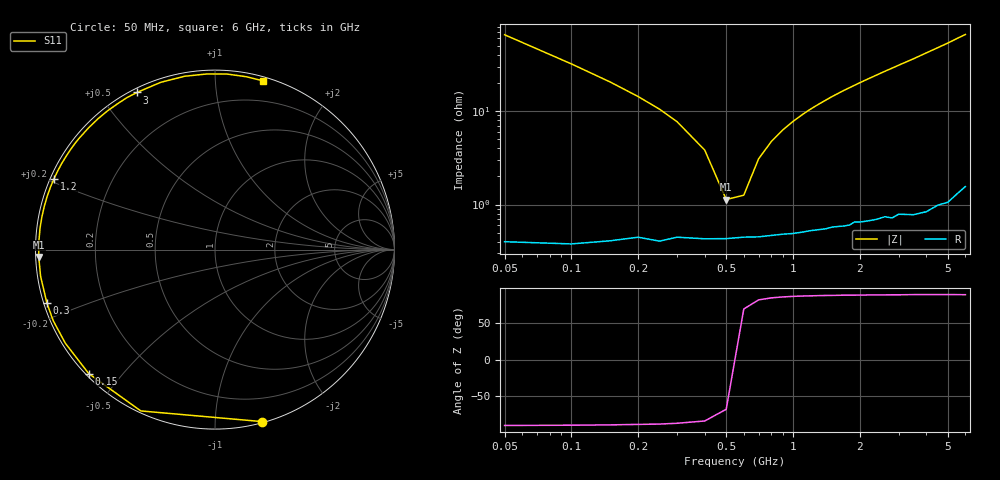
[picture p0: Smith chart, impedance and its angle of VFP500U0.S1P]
! Infineon Technologies  Discrete & RF Semiconductors
! BBY 58-03
! Si Tuning Diode in SOD323
! VR = 0.5 V
! S-Parameters:  June  1999
# GHz  S  MA  R  50
!  f  S11
! GHz  MAG  ANG
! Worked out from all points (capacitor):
!   34 points, 50 MHz to 6 GHz, reference 50 ohm
!   read as one part to ground: C = 48 pF near 50 MHz
!   lowest |Z| = 1.13 ohm at 500 MHz (marker M1)
!   series resonance near 547.1 MHz, so ESL is about 1.8 nH
!   S11 on the Smith chart (normalised r, x): 50 MHz: 0.01, -1.31; 150 MHz: 0.01, -0.41; 300 MHz: 0.01, -0.15; 1.2 GHz: 0.01, +0.21; 3 GHz: 0.02, +0.62; 6 GHz: 0.03, +1.32
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0.05  0.9941 -74.6
0.1  0.9893 -114.7
0.15  0.986 -135.5
0.2  0.9836 -148.0
0.25  0.9845 -156.3
0.3  0.9827 -162.5
0.4  0.983 -171.3
0.5  0.9829 -177.6
0.6  0.9822 177.3
0.7  0.9822 173.0
0.8  0.9816 169.2
1  0.981 162.4
1.2  0.98 156.3
1.4  0.9796 150.8
1.6  0.9789 145.6
1.7  0.979 143.1
2  0.9779 136.2
2.2  0.9778 131.9
2.4  0.9777 127.8
2.6  0.9772 123.8
2.8  0.9786 120.1
3  0.9775 116.4
3.5  0.9798 108.0
4  0.9805 99.9
4.5  0.9796 92.7
5  0.9804 86.1
5.5  0.9788 79.7
6  0.9775 74.2
